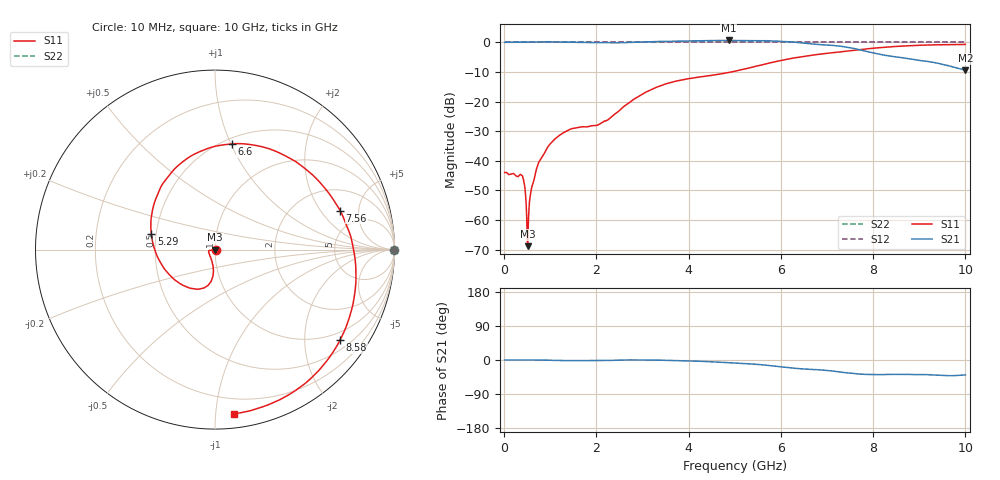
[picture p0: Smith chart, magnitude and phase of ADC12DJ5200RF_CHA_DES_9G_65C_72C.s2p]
! Texas Instruments, Inc.
! ADC12DJ5200RF - CH A S-Parameters (DES Mode, Fs = 9 GSPS, 65 degC case, 72 degC juntion)
! Port 1 represents the 100-ohm differenal input, Port 2 the digital output
! freq  dbS11  angS11  dbS21 angS21 dbS12 angS12 dbS22 angS22
# HZ S DB R 100
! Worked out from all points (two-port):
!   1000 points, 10 MHz to 10 GHz, reference 100 ohm
!   highest |S21| = 0.64 dB at 4.87 GHz (marker M1); lowest = -9.4 dB at 10 GHz (marker M2)
!   |S21| within 3 dB of the highest: start of sweep to 7.665 GHz
!   lowest |S11| = -68.9 dB at 510 MHz (marker M3), VSWR 1.00, Z = 100 - j0.0713 ohm
!   |S11| at or under -10 dB: start of sweep to 4.932 GHz
!   |S22| runs from 0.0 to 0.0 dB; largest |S21 - S12| = 0.77
!   S11 on the Smith chart (normalised r, x): 10 MHz: 1.01, -0.00; 5.29 GHz: 0.47, +0.10; 6.6 GHz: 0.55, +1.01; 7.56 GHz: 3.35, +3.13; 8.58 GHz: 0.75, -2.91; 10 GHz: 0.09, -1.12
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1e7  -43.98 -7.6  0.00 0.0  0.00 0.0  0.00 0.0
3.8e8  -44.92 -10.5  0.06 0.1  0.00 0.0  0.00 0.0
4.3e8  -47.24 -0.5  0.06 0.0  0.00 0.0  0.00 0.0
4.7e8  -52.81 6.8  0.07 -0.0  0.00 0.0  0.00 0.0
5.1e8  -68.87 -81.6  0.08 -0.0  0.00 0.0  0.00 0.0
7.1e8  -42.37 -157.4  0.10 -0.1  0.00 0.0  0.00 0.0
9.4e8  -35.52 -169.1  0.15 -0.6  0.00 0.0  0.00 0.0
1.26e9  -30.80 -171.7  0.11 -1.4  0.00 0.0  0.00 0.0
1.68e9  -28.56 -163.4  -0.03 -1.6  0.00 0.0  0.00 0.0
2.24e9  -26.25 -119.8  -0.12 -1.2  0.00 0.0  0.00 0.0
3.34e9  -14.98 -96.9  0.28 -0.3  0.00 0.0  0.00 0.0
4.19e9  -11.81 -123.4  0.55 -3.0  0.00 0.0  0.00 0.0
4.87e9  -10.20 -164.6  0.64 -7.1  0.00 0.0  0.00 0.0
5.01e9  -9.74 -174.4  0.61 -8.1  0.00 0.0  0.00 0.0
5.29e9  -8.74 165.9  0.56 -10.0  0.00 0.0  0.00 0.0
5.9e9  -6.49 126.2  0.42 -16.6  0.00 0.0  0.00 0.0
6.6e9  -4.49 81.1  -0.41 -24.4  0.00 0.0  0.00 0.0
6.67e9  -4.33 76.5  -0.53 -25.0  0.00 0.0  0.00 0.0
7.56e9  -2.73 17.4  -1.99 -35.6  0.00 0.0  0.00 0.0
8.34e9  -1.56 -25.8  -4.57 -38.0  0.00 0.0  0.00 0.0
8.58e9  -1.31 -35.9  -5.07 -37.8  0.00 0.0  0.00 0.0
1e10  -0.71 -83.2  -9.44 -39.4  0.00 0.0  0.00 0.0
